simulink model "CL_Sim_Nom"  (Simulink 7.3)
settings: Solver=ode5  StartTime=0.0  StopTime=40  FixedStep=0.02  RelTol=1e-3
InitFcn:
  | run
StopFcn:
  | Pl
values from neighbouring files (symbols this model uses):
  Afc = [    [fcs.m]
  Bfc = [    [fcs.m]
  Cfc = [    [fcs.m]
  d2r = pi/180    (= 0.0174532925199)    [run.m]
  Dfc = [    [fcs.m]
  LBThrust = 0.96097e+6    (= 960970)    [run.m]
undefined symbols (not defined in the file or in its folder): Av1, Bv1, Cv1, Dv1, nu, nuf, nx, nxf, ThVC

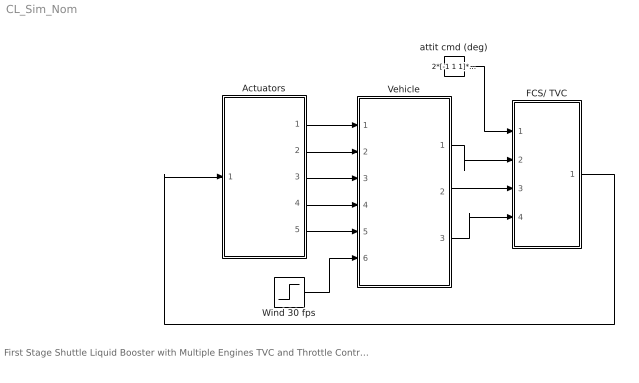
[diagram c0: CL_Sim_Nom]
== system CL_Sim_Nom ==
  note: First Stage Shuttle Liquid Booster with Multiple Engines TVC and Throttle Control Simulation Model CL_Sim_Nom.Mdl
  Actuators : Subsystem
  FCS/ TVC : Subsystem
  Vehicle : Subsystem
  Wind 30 fps : Step  Time=0  After=30  SampleTime=0
  attit cmd (deg) : Constant  Value=2*[-1 1 1]*d2r  OutDataType=sfix(16)  OutScaling=2^0
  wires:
  FCS/ TVC/1(TVC) -> Actuators/1(TVC)
  Vehicle/1(atti) -> FCS/ TVC/2(atti)
  Vehicle/2(rate) -> FCS/ TVC/3(rate)
  Vehicle/3(accel) -> FCS/ TVC/4(accel)
  Wind 30 fps/1 -> Vehicle/6(Gust)
  attit cmd (deg)/1 -> FCS/ TVC/1(atti-cmd)
  Actuators/5(DThrottle) -> Vehicle/5(Dthro)
  Actuators/3(dz (yaw)) -> Vehicle/3(dz)
  Actuators/1(dy (pitch)) -> Vehicle/1(dy)
  Actuators/4(dzdd) -> Vehicle/4(dzdd)
  Actuators/2(dydd) -> Vehicle/2(dydd)

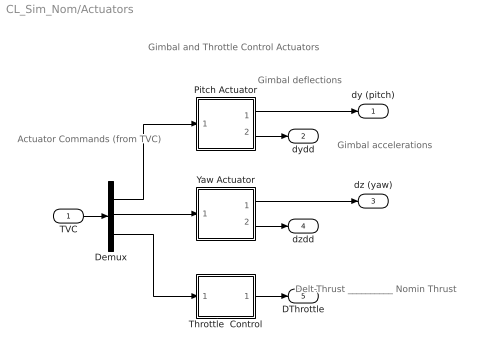
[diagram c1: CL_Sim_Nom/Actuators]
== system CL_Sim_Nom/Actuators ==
  note: Gimbal and Throttle Control Actuators
  note: Actuator Commands (from TVC)
  note: Gimbal deflections
  note: Delt-Thrust __________ Nomin Thrust
  note: Gimbal accelerations
  TVC : Inport  OutDataType=sfix(16)  OutScaling=2^0
  Demux : Demux  Outputs=[9, 9, 6]
  Pitch Actuator : Subsystem
  Throttle  Control : Subsystem
  Yaw Actuator : Subsystem
  dy (pitch) : Outport  OutDataType=sfix(16)  OutScaling=2^0
  dydd : Outport  Port=2  OutDataType=sfix(16)  OutScaling=2^0
  dz (yaw) : Outport  Port=3  OutDataType=sfix(16)  OutScaling=2^0
  dzdd : Outport  Port=4  OutDataType=sfix(16)  OutScaling=2^0
  DThrottle : Outport  Port=5  OutDataType=sfix(16)  OutScaling=2^0
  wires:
  Demux/3 -> Throttle  Control/1(thi)
  Demux/1 -> Pitch Actuator/1(dy-c)
  Demux/2 -> Yaw Actuator/1(dz-c)
  Pitch Actuator/1(dy) -> dy (pitch)/1
  TVC/1 -> Demux/1
  Throttle  Control/1(tho) -> DThrottle/1
  Yaw Actuator/1(dz) -> dz (yaw)/1
  Pitch Actuator/2(dydd) -> dydd/1
  Yaw Actuator/2(dzdd) -> dzdd/1

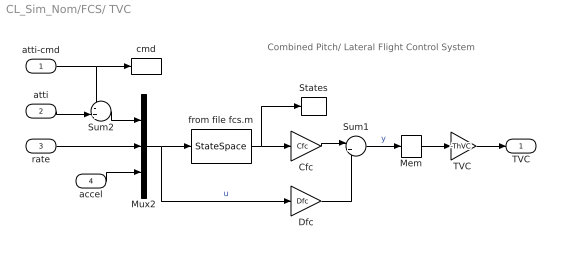
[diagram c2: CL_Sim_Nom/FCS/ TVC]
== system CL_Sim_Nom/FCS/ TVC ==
  note: Combined Pitch/ Lateral Flight Control System
  atti-cmd : Inport  OutDataType=sfix(16)  OutScaling=2^0
  atti : Inport  Port=2  OutDataType=sfix(16)  OutScaling=2^0
  rate : Inport  Port=3  OutDataType=sfix(16)  OutScaling=2^0
  accel : Inport  Port=4  OutDataType=sfix(16)  OutScaling=2^0
  Cfc : Gain  Gain=Cfc  Multiplication=Matrix(K*u)  ParameterDataType=sfix(16)  ParameterScaling=2^0  OutDataType=sfix(16)  OutScaling=2^0
  Dfc : Gain  Gain=Dfc  Multiplication=Matrix(K*u)  ParameterDataType=sfix(16)  ParameterScaling=2^0  OutDataType=sfix(16)  OutScaling=2^0
  Mem : Memory
  Mux2 : Mux  Inputs=[3, 3, 2]
  States : ToWorkspace  VariableName=xfc  SampleTime=-1  SaveFormat=Array
  Sum1 : Sum  Inputs=|++  OutDataType=sfix(16)  OutScaling=2^0
  Sum2 : Sum  Inputs=-+|  OutDataType=sfix(16)  OutScaling=2^0
  "TVC " : Gain  Gain=-ThVC  Multiplication=Matrix(K*u) (u vector)  ParameterDataType=sfix(16)  ParameterScaling=2^0  OutDataType=sfix(16)  OutScaling=2^0
  cmd : ToWorkspace  VariableName=cmd  SampleTime=-1  SaveFormat=Array
  from file fcs.m : StateSpace  A=Afc  B=Bfc  C=eye(nxf,nxf)  D=zeros(nxf,nuf)
  TVC : Outport  OutDataType=sfix(16)  OutScaling=2^0
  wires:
  Mux2/1 -> from file fcs.m/1, Dfc/1  "u"
  accel/1 -> Mux2/3
  rate/1 -> Mux2/2
  "TVC "/1 -> TVC/1
  Sum2/1 -> Mux2/1
  atti/1 -> Sum2/2
  atti-cmd/1 -> Sum2/1, cmd/1
  Mem/1 -> "TVC "/1
  Cfc/1 -> Sum1/1
  Sum1/1 -> Mem/1  "y"
  Dfc/1 -> Sum1/2
  from file fcs.m/1 -> Cfc/1, States/1

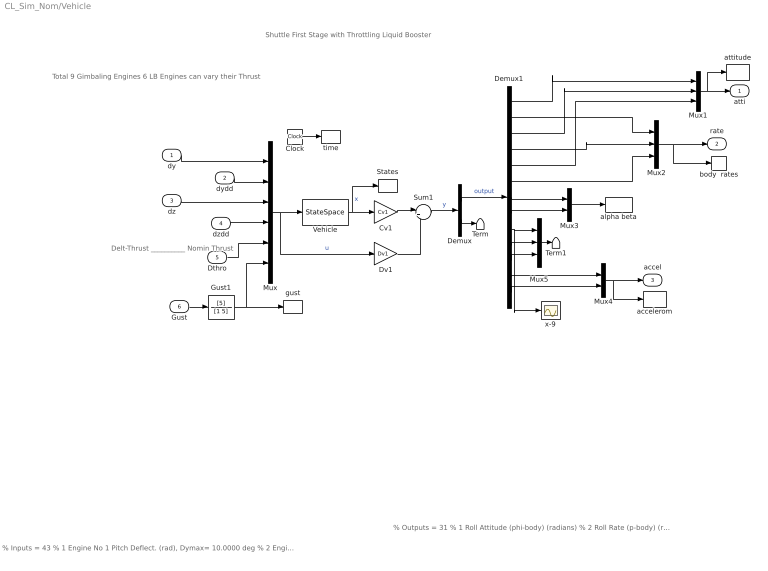
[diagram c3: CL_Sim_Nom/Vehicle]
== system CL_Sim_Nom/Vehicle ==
  note: Shuttle First Stage with Throttling Liquid Booster
  note: Total 9 Gimbaling Engines 6 LB Engines can vary their Thrust
  note: Delt-Thrust __________ Nomin Thrust
  note: % Inputs = 43 % 1 Engine No 1 Pitch Deflect. (rad), Dymax= 10.0000 deg % 2 Engine No 2 Pitch Deflect. (rad), Dymax= 10.0000 deg % 3 Engine No 3 Pitch Deflect. (rad), Dymax= 10.0000 deg % 4 Engine No 4 Pitch Deflect. (rad), Dymax= 5.0000 deg % 5 Engine No 5 Pitch Deflect. (rad), Dymax= 5.0000 deg % 6 Engine No 6 Pitch Deflect. (rad), Dymax= 5.0000 deg % 7 Engine No 7 Pitch Deflect. (rad), Dymax= 5.0000 deg % 8 Engine No 8 Pitch Deflect. (rad), Dymax= 5.0000 deg % 9 Engine No 9 Pitch Deflect. (rad), Dymax= 5.0000 deg % 10 Engine No 1 Pitch Acceleration (rad/sec^2) % 11 Engine No 2 Pitch Acceleration (rad/sec^2) % 12 Engine No 3 Pitch Acceleration (rad/sec^2) % 13 Engine No 4 Pitch Acceleration (rad/sec^2) % 14 Engine No 5 Pitch Acceleration (rad/sec^2) % 15 Engine No 6 Pitch Acceleration (rad/sec^2) % 16 Engine No 7 Pitch Acceleration (rad/sec^2) % 17 Engine No 8 Pitch Acceleration (rad/sec^2) % 18 Engine No 9 Pitch Acceleration (rad/sec^2) % 19 Engine No 1 Yaw Deflect. (rad), Dzmax= 10.0000 deg % 20 Engine No 2 Yaw Deflect. (rad), Dzmax= 10.0000 deg % 21 Engine No 3 Yaw Deflect. (rad), Dzmax= 10.0000 deg % 22 Engine No 4 Yaw Deflect. (rad), Dzmax= 1.0000 deg % 23 Engine No 5 Yaw Deflect. (rad), Dzmax= 1.0000 deg % 24 Engine No 6 Yaw Deflect. (rad), Dzmax= 1.0000 deg % 25 Engine No 7 Yaw Deflect. (rad), Dzmax= 1.0000 deg % 26 Engine No 8 Yaw Deflect. (rad), Dzmax= 1.0000 deg % 27 Engine No 9 Yaw Deflect. (rad), Dzmax= 1.0000 deg % 28 Engine No 1 Yaw Acceleration (rad/sec^2) % 29 Engine No 2 Yaw Acceleration (rad/sec^2) % 30 Engine No 3 Yaw Acceleration (rad/sec^2) % 31 Engine No 4 Yaw Acceleration (rad/sec^2) % 32 Engine No 5 Yaw Acceleration (rad/sec^2) % 33 Engine No 6 Yaw Acceleration (rad/sec^2) % 34 Engine No 7 Yaw Acceleration (rad/sec^2) % 35 Engine No 8 Yaw Acceleration (rad/sec^2) % 36 Engine No 9 Yaw Acceleration (rad/sec^2) % 37 Throttle Input dTh/Th for Engine No 4 (-) % 38 Throttle Input dTh/Th for Engine No 5 (-) % 39 Throttle Input dTh/Th for Engine No 
  note: % Outputs = 31 % 1 Roll Attitude (phi-body) (radians) % 2 Roll Rate (p-body) (rad/sec) % 3 Pitch Attitude (thet-bdy) (radians) % 4 Pitch Rate (q-body) (rad/sec) % 5 Yaw Attitude (psi-body) (radians) % 6 Yaw Rate (r-body) (rad/sec) % 7 Angle of attack, alfa, (radians) % 8 Angle of sideslip, beta, (radian) % 9 Change in Altitude, delta-h, (feet) % 10 Forward Acceleration (V-dot) (ft/sec) % 11 Cross Range Velocity (Vcr) (ft/sec) % 12 Accelerom # 1, (along Z), (ft/sec^2) Translat. Acceler % 13 Accelerom # 2, (along Y), (ft/sec^2) Translat. Acceler % 14 Ptch Load-Torque Tly for Engine: 1,(ft-lb) % 15 Ptch Load-Torque Tly for Engine: 2,(ft-lb) % 16 Ptch Load-Torque Tly for Engine: 3,(ft-lb) % 17 Ptch Load-Torque Tly for Engine: 4,(ft-lb) % 18 Ptch Load-Torque Tly for Engine: 5,(ft-lb) % 19 Ptch Load-Torque Tly for Engine: 6,(ft-lb) % 20 Ptch Load-Torque Tly for Engine: 7,(ft-lb) % 21 Ptch Load-Torque Tly for Engine: 8,(ft-lb) % 22 Ptch Load-Torque Tly for Engine: 9,(ft-lb) % 23 Yaw Load-Torque Tlz for Engine: 1,(ft-lb) % 24 Yaw Load-Torque Tlz for Engine: 2,(ft-lb) % 25 Yaw Load-Torque Tlz for Engine: 3,(ft-lb) % 26 Yaw Load-Torque Tlz for Engine: 4,(ft-lb) % 27 Yaw Load-Torque Tlz for Engine: 5,(ft-lb) % 28 Yaw Load-Torque Tlz for Engine: 6,(ft-lb) % 29 Yaw Load-Torque Tlz for Engine: 7,(ft-lb) % 30 Yaw Load-Torque Tlz for Engine: 8,(ft-lb) % 31 Yaw Load-Torque Tlz for Engine: 9,(ft-lb)
  dy : Inport  OutDataType=sfix(16)  OutScaling=2^0
  dydd : Inport  Port=2  OutDataType=sfix(16)  OutScaling=2^0
  dz : Inport  Port=3  OutDataType=sfix(16)  OutScaling=2^0
  dzdd : Inport  Port=4  OutDataType=sfix(16)  OutScaling=2^0
  Dthro : Inport  Port=5  OutDataType=sfix(16)  OutScaling=2^0
  Gust : Inport  Port=6  OutDataType=sfix(16)  OutScaling=2^0
  Clock : Clock
  Cv1 : Gain  Gain=Cv1  Multiplication=Matrix(K*u)  ParameterDataType=sfix(16)  ParameterScaling=2^0  OutDataType=sfix(16)  OutScaling=2^0
  Demux : Demux  Outputs=[13,18]
  Demux1 : Demux  Outputs=13
  Dv1 : Gain  Gain=Dv1  Multiplication=Matrix(K*u)  ParameterDataType=sfix(16)  ParameterScaling=2^0  OutDataType=sfix(16)  OutScaling=2^0
  Gust1 : TransferFcn  Numerator=[5]  Denominator=[1 5]
  Mux : Mux  Inputs=[9, 9, 9, 9, 6, 1]
  Mux1 : Mux  Inputs=3
  Mux2 : Mux  Inputs=3
  Mux3 : Mux  Inputs=2
  Mux4 : Mux  Inputs=2
  Mux5 : Mux  Inputs=3
  States : ToWorkspace  VariableName=xx  SampleTime=-1  SaveFormat=Array
  Sum1 : Sum  Inputs=|++  OutDataType=sfix(16)  OutScaling=2^0
  Term : Terminator
  Term1 : Terminator
  Vehicle : StateSpace  A=Av1  B=Bv1  C=eye(nx)  D=zeros(nx,nu)
  accelerom : ToWorkspace  VariableName=accel  SampleTime=-1  SaveFormat=Array
  alpha beta : ToWorkspace  VariableName=albet  SampleTime=-1  SaveFormat=Array
  attitude : ToWorkspace  VariableName=attit  SampleTime=-1  SaveFormat=Array
  body  rates : ToWorkspace  VariableName=wb  SampleTime=-1  SaveFormat=Array
  gust : ToWorkspace  VariableName=Gust  SampleTime=-1  SaveFormat=Array
  time : ToWorkspace  VariableName=time  SampleTime=-1  SaveFormat=Array
  x-9 : Scope
  atti : Outport  OutDataType=sfix(16)  OutScaling=2^0
  rate : Outport  Port=2  OutDataType=sfix(16)  OutScaling=2^0
  accel : Outport  Port=3  OutDataType=sfix(16)  OutScaling=2^0
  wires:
  Mux/1 -> Vehicle/1, Dv1/1  "u"
  Demux/1 -> Demux1/1  "output"
  Demux/2 -> Term/1
  Demux1/1 -> Mux1/1
  Demux1/3 -> Mux1/2
  Demux1/5 -> Mux1/3
  Demux1/2 -> Mux2/1
  Demux1/4 -> Mux2/2
  Demux1/6 -> Mux2/3
  Demux1/7 -> Mux3/1
  Demux1/8 -> Mux3/2
  Demux1/12 -> Mux4/1
  Demux1/13 -> Mux4/2
  Mux2/1 -> rate/1, body  rates/1
  Mux4/1 -> accel/1, accelerom/1
  dy/1 -> Mux/1
  dydd/1 -> Mux/2
  dz/1 -> Mux/3
  dzdd/1 -> Mux/4
  Demux1/9 -> Mux5/1, x-9/1
  Demux1/10 -> Mux5/2
  Demux1/11 -> Mux5/3
  Mux5/1 -> Term1/1
  Mux1/1 -> atti/1, attitude/1
  Gust/1 -> Gust1/1
  Gust1/1 -> Mux/6, gust/1
  Clock/1 -> time/1
  Mux3/1 -> alpha beta/1
  Vehicle/1 -> Cv1/1, States/1  "x"
  Cv1/1 -> Sum1/1
  Sum1/1 -> Demux/1  "y"
  Dv1/1 -> Sum1/2
  Dthro/1 -> Mux/5

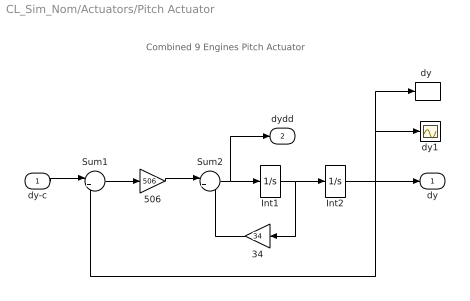
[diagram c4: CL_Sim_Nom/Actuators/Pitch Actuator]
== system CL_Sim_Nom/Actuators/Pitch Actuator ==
  note: Combined 9 Engines Pitch Actuator
  dy-c : Inport  PortDimensions=9  OutDataType=sfix(16)  OutScaling=2^0
  34 : Gain  Gain=34  ParameterDataType=sfix(16)  ParameterScaling=2^0  OutDataType=sfix(16)  OutScaling=2^0
  506 : Gain  Gain=506  ParameterDataType=sfix(16)  ParameterScaling=2^0  OutDataType=sfix(16)  OutScaling=2^0
  Int1 : Integrator
  Int2 : Integrator
  Sum1 : Sum  Inputs=|+-  OutDataType=sfix(16)  OutScaling=2^0
  Sum2 : Sum  Inputs=|+-  OutDataType=sfix(16)  OutScaling=2^0
  "dy " : ToWorkspace  VariableName=dy  SampleTime=-1  SaveFormat=Array
  dy1 : Scope
  dy : Outport  OutDataType=sfix(16)  OutScaling=2^0
  dydd : Outport  Port=2  OutDataType=sfix(16)  OutScaling=2^0
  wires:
  Sum2/1 -> Int1/1, dydd/1
  Int2/1 -> dy/1, dy1/1, "dy "/1, Sum1/2
  Int1/1 -> Int2/1, 34/1
  34/1 -> Sum2/2
  506/1 -> Sum2/1
  Sum1/1 -> 506/1
  dy-c/1 -> Sum1/1

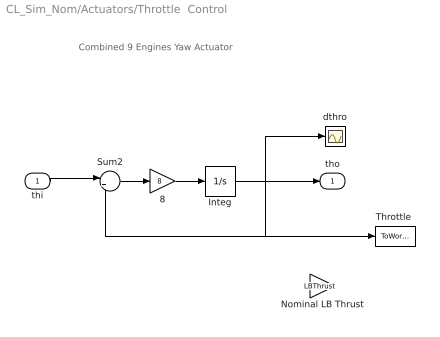
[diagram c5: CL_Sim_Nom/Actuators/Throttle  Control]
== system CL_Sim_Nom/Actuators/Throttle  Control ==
  note: Combined 9 Engines Yaw Actuator
  thi : Inport  PortDimensions=6  OutDataType=sfix(16)  OutScaling=2^0
  8 : Gain  Gain=8  ParameterDataType=sfix(16)  ParameterScaling=2^0  OutDataType=sfix(16)  OutScaling=2^0
  Integ : Integrator
  Nominal LB Thrust : Gain  Gain=LBThrust  ParameterDataType=sfix(16)  ParameterScaling=2^0  OutDataType=sfix(16)  OutScaling=2^0
  Sum2 : Sum  Inputs=|+-  OutDataType=sfix(16)  OutScaling=2^0
  "Throttle " : ToWorkspace  VariableName=Dthrust  SampleTime=-1  SaveFormat=Array
  dthro : Scope
  tho : Outport  OutDataType=sfix(16)  OutScaling=2^0
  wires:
  Sum2/1 -> 8/1
  8/1 -> Integ/1
  Integ/1 -> tho/1, dthro/1, Sum2/2, "Throttle "/1
  thi/1 -> Sum2/1

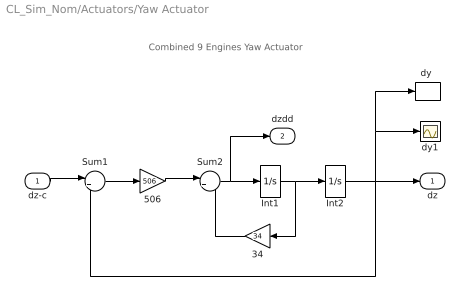
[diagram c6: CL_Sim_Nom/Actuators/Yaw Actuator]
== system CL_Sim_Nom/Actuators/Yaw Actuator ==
  note: Combined 9 Engines Yaw Actuator
  dz-c : Inport  PortDimensions=9  OutDataType=sfix(16)  OutScaling=2^0
  34 : Gain  Gain=34  ParameterDataType=sfix(16)  ParameterScaling=2^0  OutDataType=sfix(16)  OutScaling=2^0
  506 : Gain  Gain=506  ParameterDataType=sfix(16)  ParameterScaling=2^0  OutDataType=sfix(16)  OutScaling=2^0
  Int1 : Integrator
  Int2 : Integrator
  Sum1 : Sum  Inputs=|+-  OutDataType=sfix(16)  OutScaling=2^0
  Sum2 : Sum  Inputs=|+-  OutDataType=sfix(16)  OutScaling=2^0
  "dy " : ToWorkspace  VariableName=dz  SampleTime=-1  SaveFormat=Array
  dy1 : Scope
  dz : Outport  OutDataType=sfix(16)  OutScaling=2^0
  dzdd : Outport  Port=2  OutDataType=sfix(16)  OutScaling=2^0
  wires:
  Sum2/1 -> Int1/1, dzdd/1
  Int2/1 -> dz/1, dy1/1, "dy "/1, Sum1/2
  Int1/1 -> Int2/1, 34/1
  34/1 -> Sum2/2
  506/1 -> Sum2/1
  Sum1/1 -> 506/1
  dz-c/1 -> Sum1/1
